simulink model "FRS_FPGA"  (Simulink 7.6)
settings: Solver=FixedStepDiscrete  SolverMode=SingleTasking  StartTime=0.0  StopTime=6.4e-3  RelTol=1e-3
PreLoadFcn:
  | Ts_clock = 1/64e6;
libraries: dspmlti4 x8, dspsrcs4 x4, simulink x4, usrp_FPGA x1

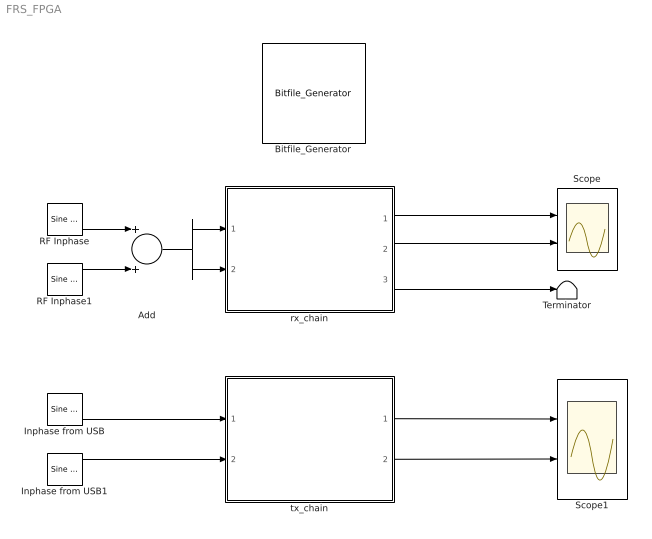
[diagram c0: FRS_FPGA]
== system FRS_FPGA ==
  Add : Sum
  Bitfile_Generator : usrp_FPGA/Bitfile_Generator  SystemSampleTime=-1
  Inphase from USB : dspsrcs4/Sine Wave  Amplitude=2^10  Frequency=200  Phase=0  SampleMode=Discrete  OutComplex=Real  CompMethod=Table lookup  TableSize=Speed  SampleTime=1/25e3  SamplesPerFrame=1  ResetState=Restart at time zero  dataType=Fixed-point  wordLen=16  udDataType=fixdt('ufix16')  fracBitsMode=User-defined  numFracBits=0  OutDataTypeStr=fixdt(1,16,0)  LastOutDataTypeStr=fixdt(1,16,0)
  Inphase from USB1 : dspsrcs4/Sine Wave  Amplitude=2^10  Frequency=5e3  Phase=0  SampleMode=Discrete  OutComplex=Real  CompMethod=Table lookup  TableSize=Speed  SampleTime=1/25e3  SamplesPerFrame=1  ResetState=Restart at time zero  dataType=Fixed-point  wordLen=16  udDataType=fixdt('ufix16')  fracBitsMode=User-defined  numFracBits=0  OutDataTypeStr=fixdt(1,16,0)  LastOutDataTypeStr=fixdt(1,16,0)
  RF Inphase : dspsrcs4/Sine Wave  Amplitude=500  Frequency=2000  Phase=0  SampleMode=Discrete  OutComplex=Real  CompMethod=Table lookup  TableSize=Speed  SampleTime=1/64e6  SamplesPerFrame=1  ResetState=Restart at time zero  dataType=Fixed-point  wordLen=16  udDataType=fixdt('fix16')  fracBitsMode=User-defined  numFracBits=0  OutDataTypeStr=fixdt(1,16,0)  LastOutDataTypeStr=fixdt(1,16,0)
  RF Inphase1 : dspsrcs4/Sine Wave  Amplitude=500  Frequency=32000  Phase=0  SampleMode=Discrete  OutComplex=Real  CompMethod=Table lookup  TableSize=Speed  SampleTime=1/64e6  SamplesPerFrame=1  ResetState=Restart at time zero  dataType=Fixed-point  wordLen=16  udDataType=fixdt('fix16')  fracBitsMode=User-defined  numFracBits=0  OutDataTypeStr=fixdt(1,16,0)  LastOutDataTypeStr=fixdt(1,16,0)
  Scope : Scope  NumInputPorts=2
  Scope1 : Scope  NumInputPorts=2
  Terminator : Terminator
  rx_chain : Subsystem
  tx_chain : Subsystem
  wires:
  rx_chain/1(i_out) -> Scope/1
  rx_chain/2(q_out) -> Scope/2
  rx_chain/3(debug) -> Terminator/1
  Inphase from USB/1 -> tx_chain/1(i_in)
  Inphase from USB1/1 -> tx_chain/2(q_in)
  tx_chain/1(i_out) -> Scope1/1
  tx_chain/2(q_out) -> Scope1/2
  RF Inphase1/1 -> Add/2
  RF Inphase/1 -> Add/1
  Add/1 -> rx_chain/1(i_in), rx_chain/2(q_in)

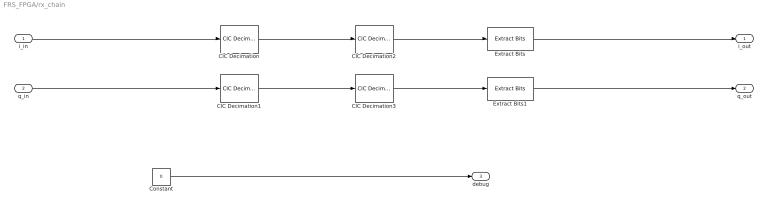
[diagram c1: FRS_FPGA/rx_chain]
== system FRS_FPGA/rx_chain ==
  i_in : Inport
  q_in : Inport  Port=2
  CIC Decimation : dspmlti4/CIC Decimation  DialogController=dspdialog.CICDecimation  filtFrom=Dialog  filtobj=CIC_decim  ftype=Decimator  R=128  M=1  N=2  filterInternals=Full precision  BPS=[2 2 2 2]  FLPS=1  outputWordLength=32  outputFracLength=1  launchFVT=off  framing=Maintain input frame rate  RateOptions=Inherit from input (this choice will be removed - see release notes)
  CIC Decimation1 : dspmlti4/CIC Decimation  DialogController=dspdialog.CICDecimation  filtFrom=Dialog  filtobj=CIC_decim  ftype=Decimator  R=128  M=1  N=2  filterInternals=Full precision  BPS=[2 2 2 2]  FLPS=1  outputWordLength=16  outputFracLength=1  launchFVT=off  framing=Maintain input frame rate  RateOptions=Inherit from input (this choice will be removed - see release notes)
  CIC Decimation2 : dspmlti4/CIC Decimation  DialogController=dspdialog.CICDecimation  filtFrom=Dialog  filtobj=CIC_decim  ftype=Decimator  R=20  M=1  N=4  filterInternals=Full precision  BPS=[2 2 2 2]  FLPS=1  outputWordLength=16  outputFracLength=1  launchFVT=off  framing=Maintain input frame rate  RateOptions=Inherit from input (this choice will be removed - see release notes)
  CIC Decimation3 : dspmlti4/CIC Decimation  DialogController=dspdialog.CICDecimation  filtFrom=Dialog  filtobj=CIC_decim  ftype=Decimator  R=20  M=1  N=4  filterInternals=Full precision  BPS=[2 2 2 2]  FLPS=1  outputWordLength=16  outputFracLength=1  launchFVT=off  framing=Maintain input frame rate  RateOptions=Inherit from input (this choice will be removed - see release notes)
  Constant : Constant  Value=0  OutDataTypeStr=boolean  SampleTime=1/64e6
  Extract Bits : simulink/Logic and Bit Operations/Extract Bits  SystemSampleTime=-1  bitsToExtract=Range starting with most significant bit  numBits=16  bitIdxRange=[0 7]  outScalingMode=Treat bit field as an integer
  Extract Bits1 : simulink/Logic and Bit Operations/Extract Bits  SystemSampleTime=-1  bitsToExtract=Range starting with most significant bit  numBits=16  bitIdxRange=[0 7]  outScalingMode=Treat bit field as an integer
  i_out : Outport
  q_out : Outport  Port=2
  debug : Outport  Port=3
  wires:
  Constant/1 -> debug/1
  CIC Decimation/1 -> CIC Decimation2/1
  CIC Decimation2/1 -> Extract Bits/1
  i_in/1 -> CIC Decimation/1
  CIC Decimation1/1 -> CIC Decimation3/1
  CIC Decimation3/1 -> Extract Bits1/1
  q_in/1 -> CIC Decimation1/1
  Extract Bits/1 -> i_out/1
  Extract Bits1/1 -> q_out/1

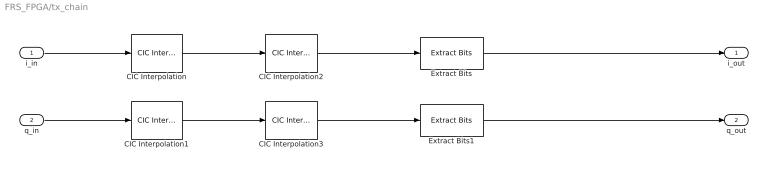
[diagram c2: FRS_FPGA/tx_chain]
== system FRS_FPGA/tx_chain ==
  i_in : Inport
  q_in : Inport  Port=2
  CIC Interpolation : dspmlti4/CIC Interpolation  DialogController=dspdialog.CICInterpolation  filtFrom=Dialog  filtobj=CIC_interp  ftype=Interpolator  R=128  M=1  N=2  filterInternals=Full precision  BPS=[16 16 16 16]  FLPS=0  outputWordLength=16  outputFracLength=0  launchFVT=off  framing=Maintain input frame size  InputProcessing=Inherited (this choice will be removed - see release notes)
  CIC Interpolation1 : dspmlti4/CIC Interpolation  DialogController=dspdialog.CICInterpolation  filtFrom=Dialog  filtobj=CIC_interp  ftype=Interpolator  R=128  M=1  N=2  filterInternals=Full precision  BPS=[16 16 16 16]  FLPS=0  outputWordLength=16  outputFracLength=0  launchFVT=off  framing=Maintain input frame size  InputProcessing=Inherited (this choice will be removed - see release notes)
  CIC Interpolation2 : dspmlti4/CIC Interpolation  DialogController=dspdialog.CICInterpolation  filtFrom=Dialog  filtobj=CIC_interp  ftype=Interpolator  R=10  M=1  N=4  filterInternals=Full precision  BPS=[16 16 16 16]  FLPS=0  outputWordLength=16  outputFracLength=0  launchFVT=off  framing=Maintain input frame size  InputProcessing=Inherited (this choice will be removed - see release notes)
  CIC Interpolation3 : dspmlti4/CIC Interpolation  DialogController=dspdialog.CICInterpolation  filtFrom=Dialog  filtobj=CIC_interp  ftype=Interpolator  R=10  M=1  N=4  filterInternals=Full precision  BPS=[16 16 16 16]  FLPS=0  outputWordLength=16  outputFracLength=0  launchFVT=off  framing=Maintain input frame size  InputProcessing=Inherited (this choice will be removed - see release notes)
  Extract Bits : simulink/Logic and Bit Operations/Extract Bits  SystemSampleTime=-1  bitsToExtract=Range starting with most significant bit  numBits=16  bitIdxRange=[0 7]  outScalingMode=Treat bit field as an integer
  Extract Bits1 : simulink/Logic and Bit Operations/Extract Bits  SystemSampleTime=-1  bitsToExtract=Range starting with most significant bit  numBits=16  bitIdxRange=[0 7]  outScalingMode=Treat bit field as an integer
  i_out : Outport
  q_out : Outport  Port=2
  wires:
  i_in/1 -> CIC Interpolation/1
  q_in/1 -> CIC Interpolation1/1
  CIC Interpolation1/1 -> CIC Interpolation3/1
  CIC Interpolation/1 -> CIC Interpolation2/1
  Extract Bits/1 -> i_out/1
  Extract Bits1/1 -> q_out/1
  CIC Interpolation2/1 -> Extract Bits/1
  CIC Interpolation3/1 -> Extract Bits1/1
